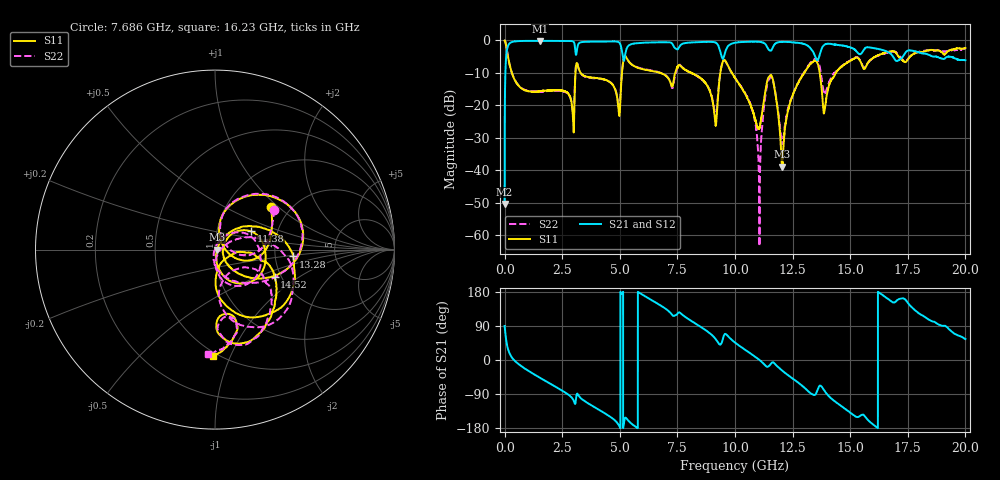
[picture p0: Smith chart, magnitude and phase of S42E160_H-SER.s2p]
! Created Wed Nov 25 22:01:19 2020
# khz S ma R 50
! 2 Port Network Data from SP1.SP block
! freq  magS11  angS11  magS21  angS21  magS12  angS12  magS22  angS22
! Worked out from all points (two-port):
!   20001 points, 300 kHz to 20 GHz, reference 50 ohm
!   highest |S21| = -0.13 dB at 1.541 GHz (marker M1); lowest = -50.4 dB at 300 kHz (marker M2)
!   |S21| within 3 dB of the highest: 97.17 MHz to 3.07 GHz (2.973 GHz wide, 188 % of centre); 5.268 GHz to 9.35 GHz (4.082 GHz wide, 55.9 % of centre)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
!   lowest |S11| = -38.9 dB at 12.05 GHz (marker M3), VSWR 1.02, Z = 51.2 - j0.0885 ohm
!   |S11| at or under -10 dB: 315.6 MHz to 3.075 GHz (2.759 GHz wide, 163 % of centre); 3.303 GHz to 5.094 GHz (1.791 GHz wide, 42.7 % of centre); 9.868 GHz to 13 GHz (3.132 GHz wide, 27.4 % of centre)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
!   |S22| runs from -63.3 to 0.0 dB; largest |S21 - S12| = 0.018
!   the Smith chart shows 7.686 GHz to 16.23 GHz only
!   S11 on the Smith chart (normalised r, x): 7.686 GHz: 1.59, +0.89; 11.38 GHz: 1.47, +0.31; 13.28 GHz: 2.54, -0.24; 14.52 GHz: 1.84, -0.65; 16.23 GHz: 0.47, -0.87
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300  0.9954 -0.3  0.003035 89.7  0.002935 90.2  0.996 -0.5
173300  0.4995 -66.2  0.8616 23.7  0.8622 23.5  0.5028 -66.1
1541300  0.1664 -135.7  0.9854 -47.2  0.984 -47.2  0.1649 -137.9
2940300  0.08991 170.9  0.9748 -101.1  0.9744 -101.1  0.09211 -171.4
3334300  0.3059 165.3  0.9416 -102.2  0.9409 -102.2  0.3027 172.5
4940300  0.09086 124.2  0.9468 -170.0  0.946 -170.0  0.1005 130.9
5237300  0.5764 141.5  0.6205 -152.2  0.622 -152.3  0.5763 138.6
6667300  0.3227 62.4  0.9364 147.6  0.9345 147.6  0.3263 55.3
7686300  0.3899 37.3  0.8758 121.0  0.8736 121.2  0.3948 34.3
9139300  0.05575 3.4  0.9317 56.9  0.9356 56.8  0.07028 14.8
9483300  0.4826 29.2  0.5225 58.0  0.5212 58.4  0.4799 30.6
1.00003e7  0.2662 -36.7  0.9213 46.1  0.921 46.2  0.2655 -45.0
1.10483e7  0.04474 5.9  0.9506 0.6  0.9529 0.7  0.005456 -116.8
1.13823e7  0.2261 26.7  0.8097 -17.8  0.8078 -17.7  0.1991 25.6
1.20473e7  0.01141 -4.3  0.9503 -28.0  0.9536 -28.2  0.02583 -30.2
1.32753e7  0.4386 -5.0  0.7587 -87.5  0.7596 -87.5  0.4534 -16.7
1.33343e7  0.4511 -12.2  0.7112 -89.8  0.7149 -89.7  0.4727 -22.5
1.38823e7  0.08014 -33.1  0.8583 -80.9  0.8606 -80.8  0.1514 -58.6
1.45183e7  0.365 -24.7  0.8491 -117.6  0.8498 -117.2  0.3707 -34.2
1.62263e7  0.5951 -91.0  0.7386 179.0  0.7352 179.3  0.5854 -93.9
1.66673e7  0.6665 -108.2  0.6582 160.1  0.643 160.1  0.6604 -117.0
2e7  0.7683 150.5  0.4943 55.1  0.4953 56.2  0.7489 144.9
